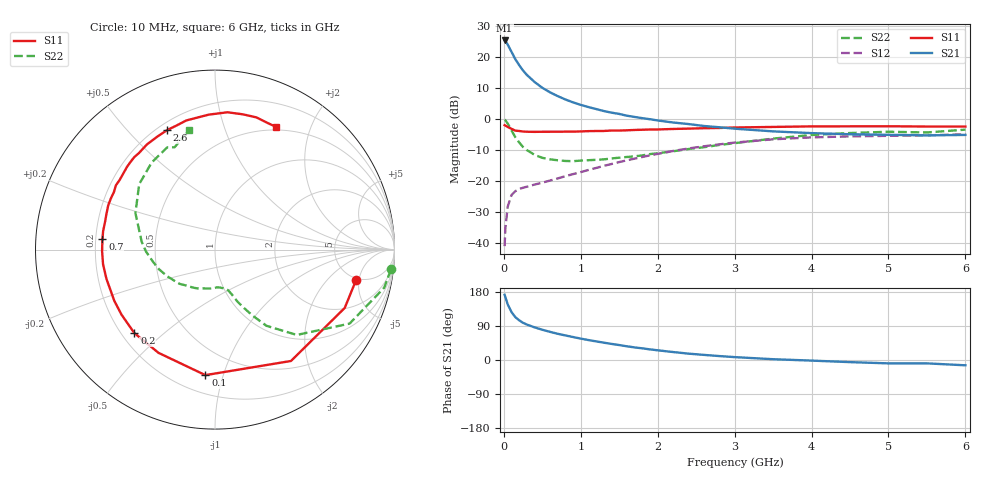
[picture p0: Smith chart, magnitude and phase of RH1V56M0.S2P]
! SIEMENS Small Signal Semiconductors
! BFR106
! Si NPN RF Bipolar Junction Transistor in SOT23
! VCE = 1.5 V  IC = 6 mA
! Common Emitter S-Parameters:  August  1996
# GHz  S  MA  R  50
!  f  S11  S21  S12  S22
! GHz  MAG  ANG  MAG  ANG  MAG  ANG  MAG  ANG
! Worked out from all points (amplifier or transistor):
!   36 points, 10 MHz to 6 GHz, reference 50 ohm
!   highest |S21| = 25.5 dB at 10 MHz (marker M1)
!   |S21| within 3 dB of that: start of sweep to 85.26 MHz
!   unconditionally stable (mu >= 1): 570.1 MHz to 2.364 GHz; 4.092 GHz to end of sweep
!   at 250 MHz: K = 0.57, MSG = 18.9 dB, |S12| = -22.1 dB
!   at 1.4 GHz: K = 1.15, MAG = 5.9 dB, |S12| = -14.4 dB
!   at 6 GHz: K = 1.03, MAG = -1.1 dB, |S12| = -4.8 dB
!   S11 on the Smith chart (normalised r, x): 10 MHz: 4.73, -4.55; 100 MHz: 0.32, -0.87; 200 MHz: 0.25, -0.40; 700 MHz: 0.23, +0.04; 2.6 GHz: 0.24, +0.65; 6 GHz: 0.46, +1.51
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0.01  0.8041 -12.2  18.81 172.1  0.0089 84.8  0.9869 -6.4
0.02  0.7926 -24.2  18.49 165.8  0.0174 78.7  0.9663 -12.7
0.05  0.7512 -55.7  16.14 147.0  0.0386 63.0  0.8558 -28.8
0.1  0.7014 -94.4  12.28 126.4  0.0599 48.2  0.6587 -46.2
0.15  0.6557 -118.7  9.343 112.9  0.069 40.2  0.5119 -56.0
0.2  0.6467 -134.0  7.482 104.7  0.0748 37.4  0.4218 -60.4
0.25  0.6345 -145.2  6.133 98.1  0.0784 36.2  0.3564 -64.0
0.3  0.6294 -153.1  5.205 93.5  0.0813 36.8  0.3179 -66.5
0.4  0.6263 -164.9  4.004 86.1  0.0882 38.6  0.2659 -69.5
0.5  0.6291 -172.5  3.23 79.8  0.0946 41.2  0.2383 -72.0
0.6  0.6292 -179.3  2.732 74.3  0.1023 43.9  0.2253 -75.3
0.7  0.6298 174.7  2.371 69.2  0.1108 46.5  0.2176 -79.5
0.9  0.6316 166.1  1.876 60.6  0.13 50.3  0.2106 -87.0
1.1  0.6438 157.6  1.576 52.6  0.1518 53.0  0.2182 -96.5
1.3  0.6477 150.5  1.36 45.7  0.1768 54.2  0.2251 -106.1
1.6  0.6638 140.4  1.143 36.1  0.2172 54.3  0.246 -121.2
2.2  0.698 122.9  0.888 21.0  0.3075 49.0  0.3039 -150.5
2.6  0.7173 111.8  0.78 13.5  0.3661 43.0  0.3536 -169.4
3.5  0.7526 92.7  0.638 2.1  0.4749 27.2  0.4876 155.4
4.5  0.7695 78.3  0.573 -5.6  0.5292 10.2  0.5999 126.0
5.5  0.7637 67.1  0.55 -8.9  0.55 0.2  0.6128 111.6
6  0.7636 63.6  0.559 -14.0  0.573 -7.1  0.6806 102.3
